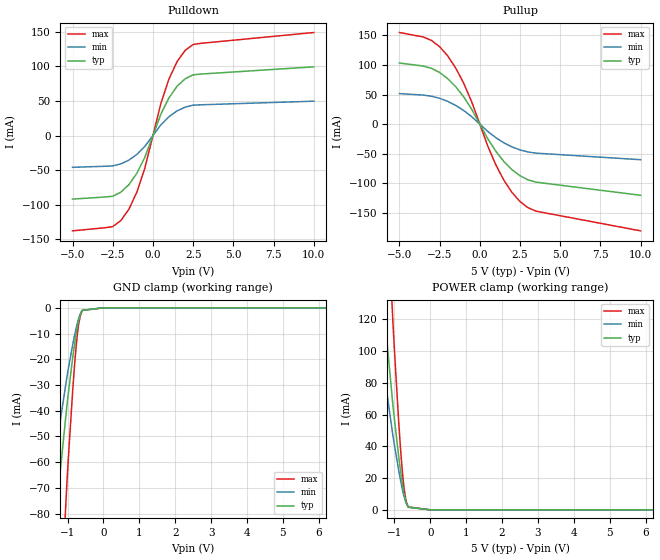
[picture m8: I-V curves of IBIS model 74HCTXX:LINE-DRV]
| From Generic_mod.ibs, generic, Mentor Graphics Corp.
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[Model]   74HCTXX:LINE-DRV
Model_type   I/O
Polarity   Non-Inverting
Vinl  =   0.800V
Vinh  =   2.000V
Vmeas =   1.500V
Cref  =  50.000pF
Rref  =   1.000kOhm
Vref  =   0.000V
|   typ   min   max
C_comp   10.000pF   5.000pF   15.000pF
[Voltage Range]   5.000V   4.500V   5.500V
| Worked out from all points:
|   slope of the pulldown table from 0 to 0.75 V, typ, clamps not added: 17.5 ohm
|   slope of the pullup table from 0 to 0.75 V, typ, clamps not added: 21.1 ohm
|   GND clamp passes 1 mA (typ) near -0.59 V on its own axis
[Pulldown]
| Voltage   I(typ)   I(min)   I(max)
-5V       -91.98mA   -45.99mA   -138mA
-2.5V     -87.88mA   -43.94mA   -131.8mA
-2V       -82.09mA   -41.04mA   -123.1mA
-1.5V     -71.3mA    -35.65mA   -106.9mA
-1V       -54.66mA   -27.33mA   -81.99mA
-500mV    -31.25mA   -15.62mA   -46.88mA
500mV     31.25mA    15.62mA    46.88mA
1V        54.66mA    27.33mA    81.99mA
1.5V      71.3mA     35.65mA    106.9mA
2V        82.09mA    41.04mA    123.1mA
3V        89.01mA    44.51mA    133.5mA
10V       99.42mA    49.71mA    149.1mA
[Pullup]
| Voltage   I(typ)   I(min)   I(max)
-5V       103.3mA    51.67mA    155mA
-3V       94.33mA    47.17mA    141.5mA
-2V       77.06mA    38.53mA    115.6mA
-1.5V     63.35mA    31.67mA    95.02mA
-1V       46.05mA    23.03mA    69.08mA
-500mV    25mA       12.5mA     37.5mA
500mV     -25mA      -12.5mA    -37.5mA
1V        -46.05mA   -23.03mA   -69.08mA
1.5V      -63.35mA   -31.67mA   -95.02mA
2.5V      -87.34mA   -43.67mA   -131mA
3.5V      -98.19mA   -49.09mA   -147.3mA
10V       -120.4mA   -60.21mA   -180.6mA
[GND Clamp]
| Voltage   I(typ)   I(min)   I(max)
-5V       -588mA     -393.8mA   -1.167A
-1.02V    -38.05mA   -26.93mA   -68.17mA
-968.2mV  -31.82mA   -22.74mA   -55.96mA
-858.7mV  -19.51mA   -14.39mA   -32.21mA
-806.5mV  -14.2mA    -10.74mA   -22.28mA
-759.2mV  -9.907mA   -7.73mA    -14.57mA
-719.6mV  -6.803mA   -5.5mA     -9.321mA
-662.8mV  -3.401mA   -2.936mA   -4.137mA
-637.9mV  -2.352mA   -2.094mA   -2.721mA
-585.6mV  -961.8uA   -907uA     -1.027mA
0V        0A         0A         0A
10V       0A         0A         0A
[POWER Clamp]
| Voltage   I(typ)   I(min)   I(max)
-5V       1.022A     684.7mA    2.028A
-1.047V   66.57mA    47.12mA    119.2mA
-994.7mV  55.66mA    39.78mA    97.89mA
-885.4mV  34.14mA    25.18mA    56.36mA
-833.1mV  24.85mA    18.79mA    38.99mA
-785.9mV  17.34mA    13.53mA    25.49mA
-746.2mV  11.9mA     9.624mA    16.31mA
-689.4mV  5.952mA    5.137mA    7.241mA
-664.5mV  4.116mA    3.665mA    4.762mA
-612.2mV  1.683mA    1.587mA    1.798mA
0V        0A         0A         0A
10V       0A         0A         0A
[Ramp]
|   typ   min   max
dV/dt_r   2.016V/3.300ns   1.273V/5.940ns   2.525V/2.420ns
dV/dt_f   2.115V/3.300ns   1.292V/5.940ns   2.631V/2.420ns
R_load =  50.000Ohm
|------------------- End of 74HCTXX:LINE-DRV ----------------------------------
